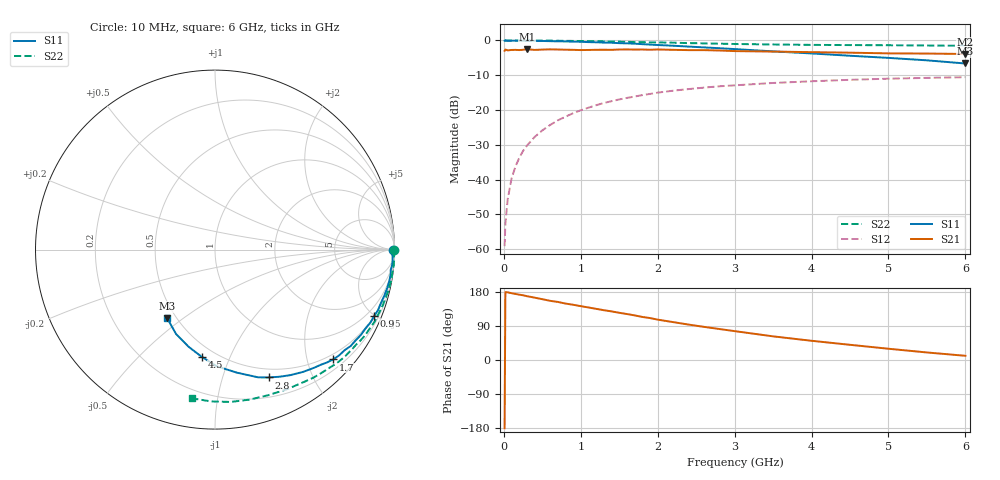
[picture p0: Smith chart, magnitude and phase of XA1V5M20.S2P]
! SIEMENS Discrete & RF Semiconductors
! BFY180
! Si NPN RF Bipolar Junction Transistor in MICRO-X
! VCE = 1.5 V  IC = 0.2 mA
! Common Emitter S-Parameters:  May  1997
# GHz  S  MA  R  50
!  f  S11  S21  S12  S22
! GHz  MAG  ANG  MAG  ANG  MAG  ANG  MAG  ANG
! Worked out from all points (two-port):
!   36 points, 10 MHz to 6 GHz, reference 50 ohm
!   highest |S21| = -2.52 dB at 300 MHz (marker M1); lowest = -3.9 dB at 6 GHz (marker M2)
!   |S21| within 3 dB of the highest: start of sweep to end of sweep
!   lowest |S11| = -6.6 dB at 6 GHz (marker M3), VSWR 2.75, Z = 22.4 - j21.9 ohm
!   |S11| at or under -10 dB: nowhere
!   |S22| runs from -1.5 to 0.0 dB; largest |S21 - S12| = 0.75
!   S11 on the Smith chart (normalised r, x): 10 MHz: open; 900 MHz: 0.51, -4.95; 1.7 GHz: 0.39, -2.49; 2.8 GHz: 0.40, -1.43; 4.5 GHz: 0.42, -0.79; 6 GHz: 0.45, -0.44
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0.01  0.992 -0.1  0.71 -180.0  0.0011 87.6  0.9997 -0.2
0.02  0.9985 -0.5  0.741 178.9  0.0023 97.1  0.9999 -0.4
0.05  0.9864 -1.2  0.72 178.6  0.0052 85.9  0.9999 -1.1
0.1  0.99 -2.3  0.73 176.3  0.0103 86.9  0.9983 -2.1
0.15  0.9916 -3.9  0.732 174.4  0.0153 86.5  0.9999 -3.1
0.2  0.9903 -5.0  0.727 172.4  0.0204 85.8  0.9994 -4.1
0.3  0.9885 -7.6  0.748 168.4  0.0307 83.0  0.9973 -6.1
0.4  0.9871 -10.2  0.731 164.6  0.0409 81.4  0.9967 -8.1
0.5  0.9826 -12.9  0.739 160.5  0.0509 78.8  0.996 -10.2
0.7  0.9713 -17.8  0.741 153.3  0.0708 74.1  0.9907 -14.3
0.9  0.9612 -22.6  0.733 145.8  0.0898 70.0  0.9851 -18.3
1.1  0.9469 -27.6  0.73 138.6  0.1079 65.6  0.9776 -22.2
1.3  0.9323 -33.0  0.735 131.4  0.1259 61.2  0.9698 -26.2
1.7  0.8991 -42.9  0.74 117.7  0.156 53.0  0.9482 -33.9
2  0.8597 -49.9  0.742 106.5  0.1776 47.3  0.9378 -39.2
2.2  0.8398 -54.2  0.733 100.0  0.1894 43.2  0.9286 -42.9
2.8  0.7735 -67.0  0.717 81.8  0.2191 33.2  0.8996 -52.5
3.5  0.6964 -79.9  0.692 62.4  0.2447 23.0  0.8752 -62.8
4  0.6505 -89.1  0.679 50.7  0.2588 16.2  0.8637 -69.9
4.5  0.6027 -96.9  0.667 40.1  0.2716 10.1  0.8577 -77.0
5.5  0.5177 -114.8  0.648 19.9  0.2896 -1.8  0.8462 -91.4
6  0.4663 -124.8  0.639 11.1  0.2964 -7.9  0.8386 -98.6
